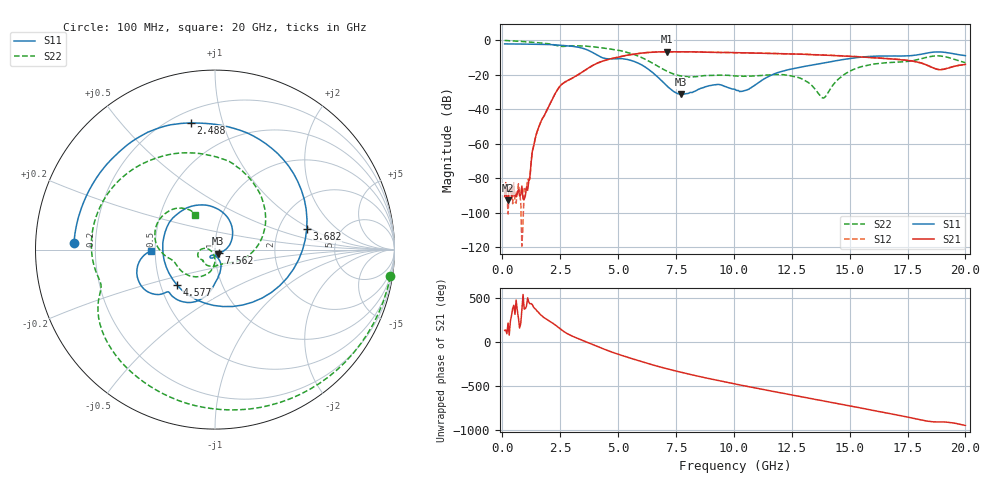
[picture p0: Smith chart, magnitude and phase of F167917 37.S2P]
!  2-Port S-parameters saved by WinCal
! VAR MeasName=S-Parameters (CALIBRATED_DATA) read from VNA (N5242A)
! VAR MeasDate=2016-11-22 9:01:36
! VAR NAME=F167917 37
! VAR FILENAME=F167917 37.S2P
! VAR DATE=2016-11-22 9:01:36
! VAR PHYS_PORTS=1,2
# Hz S DB R 50
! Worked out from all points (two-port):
!   401 points, 100 MHz to 20 GHz, reference 50 ohm
!   highest |S21| = -6.65 dB at 7.115 GHz (marker M1); lowest = -92.9 dB at 249.2 MHz (marker M2)
!   |S21| within 3 dB of the highest: 5.059 GHz to 15.44 GHz (10.38 GHz wide, 101 % of centre)
!   lowest |S11| = -31.4 dB at 7.712 GHz (marker M3), VSWR 1.06, Z = 51.5 - j2.32 ohm
!   |S11| at or under -10 dB: 4.302 GHz to 15.34 GHz (11.03 GHz wide, 112 % of centre)
!   |S22| runs from -33.5 to -0.1 dB; largest |S21 - S12| = 0.0047
!   S11 on the Smith chart (normalised r, x): 100 MHz: 0.12, +0.02; 2.488 GHz: 0.27, +0.79; 3.682 GHz: 2.88, +0.90; 4.577 GHz: 0.61, -0.26; 7.562 GHz: 1.04, -0.04; 20 GHz: 0.47, -0.01
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1e8  -2.09 177.3  -90.66 129.6  -88.62 32.5  -0.10 -8.7
2.4925e8  -2.10 173.3  -92.86 -147.4  -100.76 -19.7  -0.19 -20.9
1.095e9  -2.24 150.5  -87.04 138.3  -80.58 85.4  -0.94 -84.3
1.54275e9  -2.34 137.2  -51.48 -21.0  -51.73 -20.8  -1.43 -112.6
2.488e9  -2.87 100.8  -26.69 150.1  -26.69 149.8  -3.44 -160.9
3.43325e9  -4.48 39.4  -18.59 19.7  -18.61 19.8  -3.28 162.3
3.682e9  -5.63 12.4  -16.41 -6.6  -16.41 -6.4  -3.47 150.6
4.12975e9  -8.87 -54.5  -13.13 -55.5  -13.08 -55.4  -4.09 129.6
4.5775e9  -10.76 -137.0  -11.08 -101.8  -11.02 -102.0  -4.90 108.7
5.672e9  -12.16 97.4  -8.05 162.7  -8.07 162.4  -8.15 48.7
6.7665e9  -21.97 14.6  -6.72 77.8  -6.74 77.8  -15.41 -16.7
7.11475e9  -26.51 -10.4  -6.65 53.4  -6.67 53.5  -17.94 -33.0
7.5625e9  -30.89 -45.5  -6.66 24.0  -6.68 24.0  -20.24 -50.4
7.71175e9  -31.35 -56.2  -6.66 14.6  -6.67 14.7  -20.66 -56.4
8.9555e9  -26.29 -105.7  -6.95 -59.1  -6.94 -59.1  -20.39 -103.2
1.005e10  -28.44 -119.4  -7.15 -118.6  -7.16 -118.5  -20.69 -133.9
1.149275e10  -21.03 -68.2  -7.60 167.1  -7.58 167.1  -20.13 -149.3
1.338325e10  -14.40 -90.6  -8.33 72.2  -8.27 72.6  -26.41 172.6
1.388075e10  -13.21 -94.4  -8.61 47.7  -8.53 47.9  -33.49 -133.8
1.497525e10  -10.66 -107.1  -9.32 -6.2  -9.23 -6.3  -18.14 -101.8
1.67165e10  -9.07 -133.1  -10.69 -92.9  -10.66 -93.3  -12.89 -152.5
2e10  -8.90 -178.7  -14.03 130.2  -13.99 129.5  -12.99 119.9
